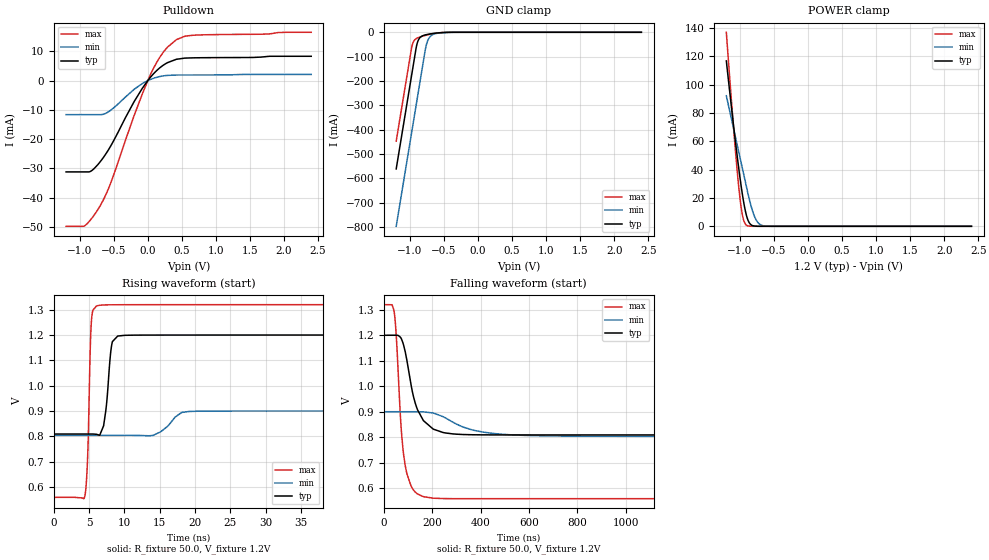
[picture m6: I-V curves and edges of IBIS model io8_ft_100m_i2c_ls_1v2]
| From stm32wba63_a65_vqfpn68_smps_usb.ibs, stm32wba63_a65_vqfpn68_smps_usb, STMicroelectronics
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[Model]   io8_ft_100m_i2c_ls_1v2
Model_type I/O_open_drain
Polarity   Non-Inverting
Enable   Active-Low
| CAP_THRESHOLD on pad IOFT is "UDTCAPC" :
| Rising=30.0% of vddiom   Falling=70.0% of vddiom
| C_comp min and max val. don't necessarily correlate with the min and max pvt
| but are the smallest and greatest pad capacitance found.
| var   typ   min   max
C_comp   2.87935pF  2.80370pF  2.98278pF
|C_comp_pulldown   2.87935pF  2.80370pF  2.98278pF
Vinl = 450.0mV
Vinh = 660.0mV
Vmeas = 600.0mV   | Reference voltage for timing measurements
Cref  = 50.0pF   | Timing specification test load capacitance value
Rref  = 1.0MOhm   | Timing specification test load resistance value
Vref  = 660.0mV   | Timing specification test load voltage
[Model Spec]
| TIME_THRESHOLD on pin ZII2CV11 is "CMOS" :
| Rising=50.0% of vdd   Falling=50.0% of vdd
Vinl 441.50000mV 335.50000mV 487.50000mV
Vinh 755.50000mV 552.50000mV 839.50000mV
| variable   typ   min   max
[Temperature Range] 25.0 140.0 -40.0
| variable   typ   min   max
[Voltage Range] 1.2V 900.0mV 1.32V
| variable   typ   min   max
[POWER Clamp Reference] 1.2V 900.0mV 1.32V
| variable   typ   min   max
[GND Clamp Reference] 0V 0V 0V
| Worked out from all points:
|   slope of the pulldown table from 0 to 0.18 V, typ, clamps not added: 40.6 ohm
|   GND clamp passes 1 mA (typ) near -0.51 V on its own axis
|   POWER clamp passes 1 mA (typ) near -0.83 V on its own axis
|   rising waveform, R_fixture 50.0, V_fixture 1.2V: 20-80 % time 730ps typ, 2.07ns min, 406ps max; typ from 0.809 V to 1.2 V
|   falling waveform, R_fixture 50.0, V_fixture 1.2V: 20-80 % time 59.8ns typ, 150ns min, 31.7ns max; typ from 1.2 V to 0.809 V
[POWER Clamp]
-1.2V     116.7mA    92.13mA    136.9mA
-1.09V    69.42mA    68.21mA    67.14mA
-1.02V    41.75mA    52.99mA    28.91mA
-990mV    30.98mA    46.47mA    16.09mA
-970mV    24.36mA    42.12mA    9.575mA
-940mV    15.59mA    35.6mA     3.485mA
-910mV    8.693mA    29.07mA    1.01mA
-860mV    2.259mA    18.59mA    104.6uA
-780mV    143.1uA    6.246mA    2.555uA
-720mV    16.22uA    1.846mA    157.1nA
-650mV    1.267uA    330.3uA    6.118nA
2.4V      0A         0A         0A
[GND Clamp]
-1.2V     -561.6mA   -797.4mA   -447.4mA
-980mV    -187.6mA   -423.4mA   -73.43mA
-960mV    -153.6mA   -389.4mA   -48.26mA
-900mV    -54.17mA   -287.4mA   -24.97mA
-870mV    -29.55mA   -236.4mA   -21.19mA
-830mV    -17.05mA   -168.4mA   -17.42mA
-760mV    -9.921mA   -54.55mA   -11.89mA
-730mV    -8.191mA   -29.78mA   -9.811mA
-690mV    -6.26mA    -14.49mA   -7.318mA
-600mV    -2.976mA   -4.315mA   -3.058mA
-380mV    -57.63uA   -251uA     -19.49uA
2.4V      872.8pA    204.8nA    349.4pA
| variable   typ   min   max
[Pullup Reference] 1.2V 900.0mV 1.32V
| variable   typ   min   max
[Pulldown Reference] 0V 0V 0V
[Pulldown]
-1.2V     -31.2mA    -11.62mA   -49.78mA
-930mV    -31.2mA    -11.62mA   -49.64mA
-830mV    -30.86mA   -11.62mA   -47.25mA
-710mV    -28.04mA   -11.62mA   -43.19mA
-550mV    -22.55mA   -10.2mA    -35.3mA
-200mV    -7.146mA   -2.964mA   -11.89mA
40mV      1.171mA    405.8uA    2.092mA
130mV     3.416mA    1.118mA    6.182mA
230mV     5.302mA    1.613mA    9.763mA
420mV     7.288mA    1.898mA    13.99mA
670mV     7.779mA    1.924mA    15.51mA
2.4V      8.312mA    2.101mA    16.51mA
[Ramp]
dV/dt_r 234.65021mV/723.16782ps 57.87422mV/1.98662ns 456.72468mV/403.46944ps
dV/dt_f 234.65962mV/57.86034ns 57.89304mV/147.86866ns 456.73579mV/31.47118ns
R_load = 50.0
| Removed startup time: 0s 0s 0s  .
| Removed end time: 49.2ns.
[Rising Waveform]
R_fixture   = 50.0
V_fixture   = 1.2V
V_fixture_min = 900.0mV
V_fixture_max = 1.32V
0s        808.9mV    803.5mV    558.8mV
4.4ns     808.9mV    803.5mV    564.4mV
4.8ns     808.9mV    803.5mV    725.3mV
5.3ns     808.9mV    803.5mV    1.244V
6.05ns    807.8mV    803.5mV    1.315V
7.05ns    841.4mV    803.5mV    1.319V
8.15ns    1.152V     803.5mV    1.319V
9.05ns    1.196V     803.5mV    1.32V
19.1ns    1.2V       897.9mV    1.32V
49.2ns    1.2V       900mV      1.32V
| Removed startup time: 0s 0s 0s  .
| Removed end time: 1.99925us.
[Falling Waveform]
R_fixture   = 50.0
V_fixture   = 1.2V
V_fixture_min = 900.0mV
V_fixture_max = 1.32V
0s        1.2V       900mV      1.32V
43ns      1.2V       900mV      1.287V
52ns      1.2V       900mV      1.181V
73ns      1.184V     900mV      812.5mV
94.75ns   1.102V     900mV      656.8mV
128.3ns   937.4mV    900mV      585.9mV
163.3ns   864.9mV    899.3mV    566.6mV
254ns     816.7mV    875.9mV    559.1mV
530.5ns   808.9mV    809.1mV    558.8mV
1.999us   808.9mV    803.5mV    558.8mV
